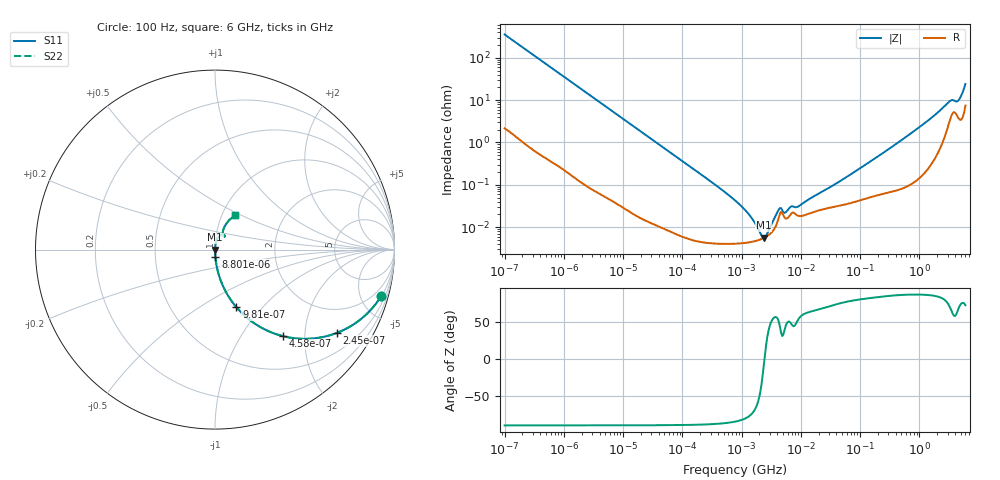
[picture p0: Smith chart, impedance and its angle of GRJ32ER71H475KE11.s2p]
!Murata Part Number: GRJ32ER71H475KE11
!These Parameters are Measured in Series Mode Connection
!Data Generated on Jun 19, 2026
!  o--ll--o
!Port1  Port2
!  o------o
!Operation Temp=25[degC], DC Bias Voltage=0[V]
!Freq. Start=100[Hz] Stop=6[GHz] 401[Steps]
# Hz S RI R 50
!Freq.(Hz) S11(Real) S11(Imag) S21(Real) S21(Imag) S12(Real) S12(Imag) S22(Real) S22(Imag)
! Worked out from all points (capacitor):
!   401 points, 100 Hz to 6 GHz, reference 50 ohm
!   read as one part in series: C = 4.46 uF near 109 Hz
!   lowest |Z| = 5.62 mohm at 2.373 MHz (marker M1)
!   series resonance near 2.436 MHz, so ESL is about 960 pH
!   S11 on the Smith chart (normalised r, x): 100 Hz: 1.04, -7.12; 245 Hz: 1.02, -2.92; 458 Hz: 1.01, -1.56; 981 Hz: 1.00, -0.73; 8.801 kHz: 1.00, -0.08; 6 GHz: 1.15, +0.46
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100  0.9255 -0.2596  0.0745 0.2596  0.0745 0.2596  0.9255 -0.2596
245  0.6794 -0.4639  0.3206 0.4639  0.3206 0.4639  0.6794 -0.4639
458  0.3795 -0.4824  0.6205 0.4824  0.6205 0.4824  0.3795 -0.4824
981  0.1196 -0.3214  0.8804 0.3214  0.8804 0.3214  0.1196 -0.3214
2008  0.0321 -0.1733  0.9679 0.1733  0.9679 0.1733  0.0321 -0.1733
8801  0.00201 -0.0411  0.998 0.0411  0.998 0.0411  0.00201 -0.0411
40335  0.000185 -0.00904  0.9998 0.00904  0.9998 0.00904  0.000185 -0.00904
774597  4.08e-05 -0.000428  1 0.000428  1 0.000428  4.08e-05 -0.000428
1212075  4.29e-05 -0.00023  1 0.00023  1 0.00023  4.29e-05 -0.00023
1813585  4.82e-05 -9.2e-05  1 9.2e-05  1 9.2e-05  4.82e-05 -9.2e-05
2372521  5.56e-05 -8.3e-06  0.9999 8.3e-06  0.9999 8.3e-06  5.56e-05 -8.3e-06
3103719  7.16e-05 7.98e-05  0.9999 -7.98e-05  0.9999 -7.98e-05  7.16e-05 7.98e-05
4440638  0.000206 0.000194  0.9998 -0.000194  0.9998 -0.000194  0.000206 0.000194
5554849  0.00016 0.000156  0.9998 -0.000156  0.9998 -0.000156  0.00016 0.000156
6644369  0.000196 0.000225  0.9998 -0.000225  0.9998 -0.000225  0.000196 0.000225
9090158  0.000185 0.000247  0.9998 -0.000247  0.9998 -0.000247  0.000185 0.000247
1.555665e7  0.000222 0.000456  0.9998 -0.000456  0.9998 -0.000456  0.000222 0.000456
3.124326e8  0.000711 0.00712  0.9993 -0.00712  0.9993 -0.00712  0.000711 0.00712
1.309207e9  0.00303 0.0303  0.997 -0.0303  0.997 -0.0303  0.00303 0.0303
3.205649e9  0.0359 0.082  0.9641 -0.082  0.9641 -0.082  0.0359 0.082
4.385646e9  0.0464 0.0767  0.9536 -0.0767  0.9536 -0.0767  0.0464 0.0767
6e9  0.1098 0.1902  0.8902 -0.1902  0.8902 -0.1902  0.1098 0.1902
